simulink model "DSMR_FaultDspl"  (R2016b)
settings: Solver=FixedStepDiscrete  StartTime=0.0  StopTime=10.0  FixedStep=0.02  RelTol=1e-3  EnableMultiTasking=on
undefined symbols (not defined in the file): bin2dec
libraries: simulink x312
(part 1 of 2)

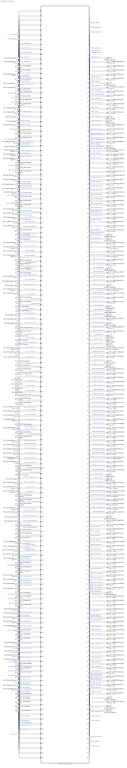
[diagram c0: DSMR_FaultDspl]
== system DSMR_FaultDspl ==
  DFC_CurrRngErr : Inport
  DFC_BattVoltRngErr : Inport  Port=2
  DFC_BattHVMsgTmt : Inport  Port=3
  DFC_BusHVMsgTmt : Inport  Port=4
  DFC_638LinCommErr : Inport  Port=5
  DFC_CellTempTmt : Inport  Port=6
  DFC_CellVoltTmt : Inport  Port=7
  DFC_InCanBusOff : Inport  Port=8
  DFC_VeCanBusOff : Inport  Port=9
  DFC_Msg2A3Tmt : Inport  Port=10
  DFC_RcMsg2A3Mis : Inport  Port=11
  DFC_ChkSumMsg2A3Err : Inport  Port=12
  DFC_RcMsg2A5Mis : Inport  Port=13
  DFC_RcMsg2A7Mis : Inport  Port=14
  DFC_CrashNpl : Inport  Port=15
  DFC_FuseNpl : Inport  Port=16
  DFC_Kl30cVoltLoErr : Inport  Port=17
  DFC_PosStuckMax : Inport  Port=18
  DFC_MPosStuckMin : Inport  Port=19
  DFC_MNegStuckMax : Inport  Port=20
  DFC_MNegStuckMin : Inport  Port=21
  DFC_PrStuckMin : Inport  Port=22
  DFC_DChrgPosStuckMax : Inport  Port=23
  DFC_DChrgPosStuckMin : Inport  Port=24
  DFC_DChrgNegStuckMax : Inport  Port=25
  DFC_DChrgNegStuckMin : Inport  Port=26
  DFC_HvPwrUpFail : Inport  Port=27
  DFC_DChrgPwrUpFail : Inport  Port=28
  DFC_BattTAlrmMax : Inport  Port=29
  DFC_BattTFaultMax : Inport  Port=30
  DFC_BattTAlrmMin : Inport  Port=31
  DFC_BattTFaultMin : Inport  Port=32
  DFC_BattTempVldMin : Inport  Port=33
  DFC_BattTCnstMax : Inport  Port=34
  DFC_BattTGradtMax : Inport  Port=35
  DFC_CellVoltAlrmMax : Inport  Port=36
  DFC_CellVoltFaultMax : Inport  Port=37
  DFC_CellVoltFusfMax : Inport  Port=38
  DFC_CellVoltAlrmMin : Inport  Port=39
  DFC_CellVoltFusfMin : Inport  Port=40
  DFC_CellVoltFaultMin : Inport  Port=41
  DFC_CellVoltVldMin : Inport  Port=42
  DFC_CellVoltNpl : Inport  Port=43
  DFC_Msg2E6Tmt : Inport  Port=44
  DFC_RcMsg2E6Mis : Inport  Port=45
  DFC_ChkSumMsg2E6Err : Inport  Port=46
  DFC_RcMsg2E1Mis : Inport  Port=47
  DFC_ChkSumMsg2E1Err : Inport  Port=48
  DFC_DcCanBusOff : Inport  Port=49
  DFC_DChrgTCnntMax : Inport  Port=50
  DFC_ChrgOCNpl : Inport  Port=51
  DFC_DisChOCNpl : Inport  Port=52
  DFC_BattVoltHiMax : Inport  Port=53
  DFC_BattVoltLoMin : Inport  Port=54
  DFC_ThmRnwy : Inport  Port=55
  DFC_AChrgPortOvrTemp : Inport  Port=56
  DFC_CurrOffsPlaus : Inport  Port=57
  DFC_CurrStukPlaus : Inport  Port=58
  DFC_CurrChrgPlaus : Inport  Port=59
  DFC_BattUNpl : Inport  Port=60
  DFC_BattVoltVld : Inport  Port=61
  DFC_PackUNpl : Inport  Port=62
  DFC_PackVoltVld : Inport  Port=63
  DFC_DChrgUNpl : Inport  Port=64
  DFC_DChrgVoltVld : Inport  Port=65
  DFC_BoardTempTmt : Inport  Port=66
  DFC_HvilMax : Inport  Port=67
  DFC_HvilMin : Inport  Port=68
  DFC_HvilSig : Inport  Port=69
  DFC_ChkSumMsg050Err : Inport  Port=70
  DFC_RcMsg050Mis : Inport  Port=71
  DFC_CrashHwNpl : Inport  Port=72
  DFC_IsoChkLv1 : Inport  Port=73
  DFC_IsoChkLv2 : Inport  Port=74
  DFC_InsResValdFault : Inport  Port=75
  DFC_Kl30OutRngErr : Inport  Port=76
  DFC_Kl30VoltLoErr : Inport  Port=77
  DFC_Kl30VoltHiErr : Inport  Port=78
  DFC_EepReadErr : Inport  Port=79
  DFC_BalStuckMax : Inport  Port=80
  DFC_BalStuckMin : Inport  Port=81
  DFC_CSCPwrSpyHiErr : Inport  Port=82
  DFC_CSCPwrSpyLoErr : Inport  Port=83
  DFC_CmcBordOTMax : Inport  Port=84
  DFC_BattTWarnMax : Inport  Port=85
  DFC_BattTWarnMin : Inport  Port=86
  DFC_BattTempVldMax : Inport  Port=87
  DFC_BattTHopMax : Inport  Port=88
  DFC_CellVoltRngHiErr : Inport  Port=89
  DFC_CellVoltRngLoErr : Inport  Port=90
  DFC_CellVoltWarnMax : Inport  Port=91
  DFC_CellVoltWarnMin : Inport  Port=92
  DFC_CellVoltVldMax : Inport  Port=93
  DFC_AChrgCurrMish : Inport  Port=94
  DFC_DChrgCurrMish : Inport  Port=95
  DFC_DChrgLowTempCurrMish : Inport  Port=96
  DFC_AChrgVoltMish : Inport  Port=97
  DFC_DChrgVoltMish : Inport  Port=98
  DFC_DChrgBattTMin : Inport  Port=99
  DFC_CC2Chk : Inport  Port=100
  DFC_APlusChk : Inport  Port=101
  DFC_DChrgMsgTmt : Inport  Port=102
  DFC_DChrgTNegElecMax : Inport  Port=103
  DFC_DChrgTNegElecMin : Inport  Port=104
  DFC_DChrgTNegElecSig : Inport  Port=105
  DFC_DChrgTPosElecMax : Inport  Port=106
  DFC_DChrgTPosElecMin : Inport  Port=107
  DFC_DChrgTPosElecSig : Inport  Port=108
  DFC_CcuSelfChkErr : Inport  Port=109
  DFC_ChrgOCMin : Inport  Port=110
  DFC_ChrgOCMax : Inport  Port=111
  DFC_DisChOCMin : Inport  Port=112
  DFC_DisChOCMax : Inport  Port=113
  DFC_SocRngLoMax : Inport  Port=114
  DFC_SocRngLoMin : Inport  Port=115
  DFC_SocRngHiMax : Inport  Port=116
  DFC_SocRngHiMin : Inport  Port=117
  DFC_InClntOverTmp : Inport  Port=118
  DFC_OutClntOverTmp : Inport  Port=119
  DFC_ClntDsTElecMax : Inport  Port=120
  DFC_ClntDsTElecMin : Inport  Port=121
  DFC_ClntDsTElecSig : Inport  Port=122
  DFC_ClntUsTElecMax : Inport  Port=123
  DFC_ClntUsTElecMin : Inport  Port=124
  DFC_ClntUsTElecSig : Inport  Port=125
  DFC_CoolPerfPlaus : Inport  Port=126
  DFC_HtgPerfPlaus : Inport  Port=127
  DFC_DChrgFobd : Inport  Port=128
  DFC_DChrgHvOnFail : Inport  Port=129
  DFC_AChgHVOnTmt : Inport  Port=130
  DFC_AChgHVOffTmt : Inport  Port=131
  DFC_AChgS2ClsdTmt : Inport  Port=132
  DFC_DChrgStakeErr : Inport  Port=133
  DFC_DChrgStkVoltErr : Inport  Port=134
  DFC_DChrgStkCurrErr : Inport  Port=135
  DFC_AChgPileRdyTmt : Inport  Port=136
  DFC_DChrgCHMTmt : Inport  Port=137
  DFC_DChrgCRMTmt : Inport  Port=138
  DFC_DChrgCMLTmt : Inport  Port=139
  DFC_DChrgCROTmt : Inport  Port=140
  DFC_DChrgCCSTmt : Inport  Port=141
  DFC_DChrgCSTTmt : Inport  Port=142
  DFC_DChrgCSDTmt : Inport  Port=143
  DFC_DChrgParaChk : Inport  Port=144
  DFC_DChrgCableChk : Inport  Port=145
  DFC_DChrgSLACTOut : Inport  Port=146
  DFC_DChrgCnntErr : Inport  Port=147
  DFC_DChrgLckErr : Inport  Port=148
  DFC_AChrgCnntErr : Inport  Port=149
  DFC_AChgLckTmt : Inport  Port=150
  DFC_AChgRdyPndiTmt : Inport  Port=151
  DFC_AChgRdyTmt : Inport  Port=152
  DFC_AChgingErr : Inport  Port=153
  DFC_AChgUnlckTmt : Inport  Port=154
  DFC_AChgFobd : Inport  Port=155
  DFC_SocValJmp : Inport  Port=156
  BMS_DSMR_FaultDspl : Subsystem
  DSMR_CurrRngErr : Outport
  DSMR_BattVoltRngErr : Outport  Port=2
  DSMR_BattHVMsgTmt : Outport  Port=3
  DSMR_BusHVMsgTmt : Outport  Port=4
  DSMR_638LinCommErr : Outport  Port=5
  DSMR_CellTempTmt : Outport  Port=6
  DSMR_CellVoltTmt : Outport  Port=7
  DSMR_InCanBusOff : Outport  Port=8
  DSMR_VeCanBusOff : Outport  Port=9
  DSMR_Msg2A3Tmt : Outport  Port=10
  DSMR_RcMsg2A3Mis : Outport  Port=11
  DSMR_ChkSumMsg2A3Err : Outport  Port=12
  DSMR_RcMsg2A5Mis : Outport  Port=13
  DSMR_RcMsg2A7Mis : Outport  Port=14
  DSMR_CrashNpl : Outport  Port=15
  DSMR_FuseNpl : Outport  Port=16
  DSMR_Kl30cVoltLoErr : Outport  Port=17
  DSMR_PosStuckMax : Outport  Port=18
  DSMR_MPosStuckMin : Outport  Port=19
  DSMR_MNegStuckMax : Outport  Port=20
  DSMR_MNegStuckMin : Outport  Port=21
  DSMR_PrStuckMin : Outport  Port=22
  DSMR_DChrgPosStuckMax : Outport  Port=23
  DSMR_DChrgPosStuckMin : Outport  Port=24
  DSMR_DChrgNegStuckMax : Outport  Port=25
  DSMR_DChrgNegStuckMin : Outport  Port=26
  DSMR_HvPwrUpFail : Outport  Port=27
  DSMR_DChrgPwrUpFail : Outport  Port=28
  DSMR_BattTAlrmMax : Outport  Port=29
  DSMR_BattTFaultMax : Outport  Port=30
  DSMR_BattTAlrmMin : Outport  Port=31
  DSMR_BattTFaultMin : Outport  Port=32
  DSMR_BattTempVldMin : Outport  Port=33
  DSMR_BattTCnstMax : Outport  Port=34
  DSMR_BattTGradtMax : Outport  Port=35
  DSMR_CellVoltAlrmMax : Outport  Port=36
  DSMR_CellVoltFaultMax : Outport  Port=37
  DSMR_CellVoltFusfMax : Outport  Port=38
  DSMR_CellVoltAlrmMin : Outport  Port=39
  DSMR_CellVoltFusfMin : Outport  Port=40
  DSMR_CellVoltFaultMin : Outport  Port=41
  DSMR_CellVoltVldMin : Outport  Port=42
  DSMR_CellVoltNpl : Outport  Port=43
  DSMR_Obc2E6Tmt : Outport  Port=44
  DSMR_RcMsg2E6Mis : Outport  Port=45
  DSMR_ChkSumMsg2E6Err : Outport  Port=46
  DSMR_RcMsg2E1Mis : Outport  Port=47
  DSMR_ChkSumMsg2E1Err : Outport  Port=48
  DSMR_DcCanBusOff : Outport  Port=49
  DSMR_DChrgTCnntMax : Outport  Port=50
  DSMR_ChrgOCNpl : Outport  Port=51
  DSMR_DisChOCNpl : Outport  Port=52
  DSMR_BattVoltHiMax : Outport  Port=53
  DSMR_BattVoltLoMin : Outport  Port=54
  DSMR_ThmRnwy : Outport  Port=55
  DSMR_AChrgPortOvrTemp : Outport  Port=56
  DSMR_CurrOffsPlaus : Outport  Port=57
  DSMR_CurrStukPlaus : Outport  Port=58
  DSMR_CurrChrgPlaus : Outport  Port=59
  DSMR_BattUNpl : Outport  Port=60
  DSMR_BattVoltVld : Outport  Port=61
  DSMR_PackUNpl : Outport  Port=62
  DSMR_PackVoltVld : Outport  Port=63
  DSMR_DChrgUNpl : Outport  Port=64
  DSMR_DChrgVoltVld : Outport  Port=65
  DSMR_BoardTempTmt : Outport  Port=66
  DSMR_HvilMax : Outport  Port=67
  DSMR_HvilMin : Outport  Port=68
  DSMR_HvilSig : Outport  Port=69
  DSMR_ChkSumMsg050Err : Outport  Port=70
  DSMR_RcMsg050Mis : Outport  Port=71
  DSMR_CrashHwNpl : Outport  Port=72
  DSMR_IsoChkLv1 : Outport  Port=73
  DSMR_IsoChkLv2 : Outport  Port=74
  DSMR_InsResValdFault : Outport  Port=75
  DSMR_Kl30OutRngErr : Outport  Port=76
  DSMR_Kl30VoltLoErr : Outport  Port=77
  DSMR_Kl30VoltHiErr : Outport  Port=78
  DSMR_EepReadErr : Outport  Port=79
  DSMR_BalStuckMax : Outport  Port=80
  DSMR_BalStuckMin : Outport  Port=81
  DSMR_CSCPwrSpyHiErr : Outport  Port=82
  DSMR_CSCPwrSpyLoErr : Outport  Port=83
  DSMR_CmcBordOTMax : Outport  Port=84
  DSMR_BattTWarnMax : Outport  Port=85
  DSMR_BattTWarnMin : Outport  Port=86
  DSMR_BattTempVldMax : Outport  Port=87
  DSMR_BattTHopMax : Outport  Port=88
  DSMR_CellVoltRngHiErr : Outport  Port=89
  DSMR_CellVoltRngLoErr : Outport  Port=90
  DSMR_CellVoltWarnMax : Outport  Port=91
  DSMR_CellVoltWarnMin : Outport  Port=92
  DSMR_CellVoltVldMax : Outport  Port=93
  DSMR_AChrgCurrMish : Outport  Port=94
  DSMR_DChrgCurrMish : Outport  Port=95
  DSMR_DChrgLowTempCurrMish : Outport  Port=96
  DSMR_AChrgVoltMish : Outport  Port=97
  DSMR_DChrgVoltMish : Outport  Port=98
  DSMR_DChrgBattTMin : Outport  Port=99
  DSMR_CC2Chk : Outport  Port=100
  DSMR_APlusChk : Outport  Port=101
  DSMR_DChrgMsgTmt : Outport  Port=102
  DSMR_DChrgTNegElecMax : Outport  Port=103
  DSMR_DChrgTNegElecMin : Outport  Port=104
  DSMR_DChrgTNegElecSig : Outport  Port=105
  DSMR_DChrgTPosElecMax : Outport  Port=106
  DSMR_DChrgTPosElecMin : Outport  Port=107
  DSMR_DChrgTPosElecSig : Outport  Port=108
  DSMR_CcuSelfChkErr : Outport  Port=109
  DSMR_ChrgOCMin : Outport  Port=110
  DSMR_ChrgOCMax : Outport  Port=111
  DSMR_DisChOCMin : Outport  Port=112
  DSMR_DisChOCMax : Outport  Port=113
  DSMR_SocRngLoMax : Outport  Port=114
  DSMR_SocRngLoMin : Outport  Port=115
  DSMR_SocRngHiMax : Outport  Port=116
  DSMR_SocRngHiMin : Outport  Port=117
  DSMR_InClntOverTmp : Outport  Port=118
  DSMR_OutClntOverTmp : Outport  Port=119
  DSMR_ClntDsTElecMax : Outport  Port=120
  DSMR_ClntDsTElecMin : Outport  Port=121
  DSMR_ClntDsTElecSig : Outport  Port=122
  DSMR_ClntUsTElecMax : Outport  Port=123
  DSMR_ClntUsTElecMin : Outport  Port=124
  DSMR_ClntUsTElecSig : Outport  Port=125
  DSMR_CoolPerfPlaus : Outport  Port=126
  DSMR_HtgPerfPlaus : Outport  Port=127
  DSMR_DChrgFobd : Outport  Port=128
  DSMR_DChrgHvOnFail : Outport  Port=129
  DSMR_AChgHVOnTmt : Outport  Port=130
  DSMR_AChgHVOffTmt : Outport  Port=131
  DSMR_AChgS2ClsdTmt : Outport  Port=132
  DSMR_DChrgStakeErr : Outport  Port=133
  DSMR_DChrgStkVoltErr : Outport  Port=134
  DSMR_DChrgStkCurrErr : Outport  Port=135
  DSMR_AChgPileRdyTmt : Outport  Port=136
  DSMR_DChrgCHMTmt : Outport  Port=137
  DSMR_DChrgCRMTmt : Outport  Port=138
  DSMR_DChrgCMLTmt : Outport  Port=139
  DSMR_DChrgCROTmt : Outport  Port=140
  DSMR_DChrgCCSTmt : Outport  Port=141
  DSMR_DChrgCSTTmt : Outport  Port=142
  DSMR_DChrgCSDTmt : Outport  Port=143
  DSMR_DChrgParaChk : Outport  Port=144
  DSMR_DChrgCableChk : Outport  Port=145
  DSMR_DChrgSLACTOut : Outport  Port=146
  DSMR_DChrgCnntErr : Outport  Port=147
  DSMR_DChrgLckErr : Outport  Port=148
  DSMR_AChrgCnntErr : Outport  Port=149
  DSMR_AChgLckTmt : Outport  Port=150
  DSMR_AChgRdyPndiTmt : Outport  Port=151
  DSMR_AChgRdyTmt : Outport  Port=152
  DSMR_AChgingErr : Outport  Port=153
  DSMR_AChgUnlckTmt : Outport  Port=154
  DSMR_AChgFobd : Outport  Port=155
  DSMR_SocValJmp : Outport  Port=156
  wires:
  DFC_CurrRngErr/1 -> BMS_DSMR_FaultDspl/1(DFC_CurrRngErr)  "DFC_CurrRngErr"
  DFC_BattVoltRngErr/1 -> BMS_DSMR_FaultDspl/2(DFC_BattVoltRngErr)  "DFC_BattVoltRngErr"
  DFC_BattHVMsgTmt/1 -> BMS_DSMR_FaultDspl/3(DFC_BattHVMsgTmt)  "DFC_BattHVMsgTmt"
  DFC_BusHVMsgTmt/1 -> BMS_DSMR_FaultDspl/4(DFC_BusHVMsgTmt)  "DFC_BusHVMsgTmt"
  DFC_638LinCommErr/1 -> BMS_DSMR_FaultDspl/5(DFC_638LinCommErr)  "DFC_638LinCommErr"
  DFC_CellTempTmt/1 -> BMS_DSMR_FaultDspl/6(DFC_CellTempTmt)  "DFC_CellTempTmt"
  DFC_CellVoltTmt/1 -> BMS_DSMR_FaultDspl/7(DFC_CellVoltTmt)  "DFC_CellVoltTmt"
  DFC_InCanBusOff/1 -> BMS_DSMR_FaultDspl/8(DFC_InCanBusOff)  "DFC_InCanBusOff"
  DFC_VeCanBusOff/1 -> BMS_DSMR_FaultDspl/9(DFC_VeCanBusOff)  "DFC_VeCanBusOff"
  DFC_Msg2A3Tmt/1 -> BMS_DSMR_FaultDspl/10(DFC_Msg2A3Tmt)  "DFC_Msg2A3Tmt"
  DFC_RcMsg2A3Mis/1 -> BMS_DSMR_FaultDspl/11(DFC_RcMsg2A3Mis)  "DFC_RcMsg2A3Mis"
  DFC_ChkSumMsg2A3Err/1 -> BMS_DSMR_FaultDspl/12(DFC_ChkSumMsg2A3Err)  "DFC_ChkSumMsg2A3Err"
  DFC_RcMsg2A5Mis/1 -> BMS_DSMR_FaultDspl/13(DFC_RcMsg2A5Mis)  "DFC_RcMsg2A5Mis"
  DFC_RcMsg2A7Mis/1 -> BMS_DSMR_FaultDspl/14(DFC_RcMsg2A7Mis)  "DFC_RcMsg2A7Mis"
  DFC_CrashNpl/1 -> BMS_DSMR_FaultDspl/15(DFC_CrashNpl)  "DFC_CrashNpl"
  DFC_FuseNpl/1 -> BMS_DSMR_FaultDspl/16(DFC_FuseNpl)  "DFC_FuseNpl"
  DFC_Kl30cVoltLoErr/1 -> BMS_DSMR_FaultDspl/17(DFC_Kl30cVoltLoErr)  "DFC_Kl30cVoltLoErr"
  DFC_PosStuckMax/1 -> BMS_DSMR_FaultDspl/18(DFC_PosStuckMax)  "DFC_PosStuckMax"
  DFC_MPosStuckMin/1 -> BMS_DSMR_FaultDspl/19(DFC_MPosStuckMin)  "DFC_MPosStuckMin"
  DFC_MNegStuckMax/1 -> BMS_DSMR_FaultDspl/20(DFC_MNegStuckMax)  "DFC_MNegStuckMax"
  DFC_MNegStuckMin/1 -> BMS_DSMR_FaultDspl/21(DFC_MNegStuckMin)  "DFC_MNegStuckMin"
  DFC_PrStuckMin/1 -> BMS_DSMR_FaultDspl/22(DFC_PrStuckMin)  "DFC_PrStuckMin"
  DFC_DChrgPosStuckMax/1 -> BMS_DSMR_FaultDspl/23(DFC_DChrgPosStuckMax)  "DFC_DChrgPosStuckMax"
  DFC_DChrgPosStuckMin/1 -> BMS_DSMR_FaultDspl/24(DFC_DChrgPosStuckMin)  "DFC_DChrgPosStuckMin"
  DFC_DChrgNegStuckMax/1 -> BMS_DSMR_FaultDspl/25(DFC_DChrgNegStuckMax)  "DFC_DChrgNegStuckMax"
  DFC_DChrgNegStuckMin/1 -> BMS_DSMR_FaultDspl/26(DFC_DChrgNegStuckMin)  "DFC_DChrgNegStuckMin"
  DFC_HvPwrUpFail/1 -> BMS_DSMR_FaultDspl/27(DFC_HvPwrUpFail)  "DFC_HvPwrUpFail"
  DFC_DChrgPwrUpFail/1 -> BMS_DSMR_FaultDspl/28(DFC_DChrgPwrUpFail)  "DFC_DChrgPwrUpFail"
  DFC_BattTAlrmMax/1 -> BMS_DSMR_FaultDspl/29(DFC_BattTAlrmMax)  "DFC_BattTAlrmMax"
  DFC_BattTFaultMax/1 -> BMS_DSMR_FaultDspl/30(DFC_BattTFaultMax)  "DFC_BattTFaultMax"
  DFC_BattTAlrmMin/1 -> BMS_DSMR_FaultDspl/31(DFC_BattTAlrmMin)  "DFC_BattTAlrmMin"
  DFC_BattTFaultMin/1 -> BMS_DSMR_FaultDspl/32(DFC_BattTFaultMin)  "DFC_BattTFaultMin"
  DFC_BattTempVldMin/1 -> BMS_DSMR_FaultDspl/33(DFC_BattTempVldMin)  "DFC_BattTempVldMin"
  DFC_BattTCnstMax/1 -> BMS_DSMR_FaultDspl/34(DFC_BattTCnstMax)  "DFC_BattTCnstMax"
  DFC_BattTGradtMax/1 -> BMS_DSMR_FaultDspl/35(DFC_BattTGradtMax)  "DFC_BattTGradtMax"
  DFC_CellVoltAlrmMax/1 -> BMS_DSMR_FaultDspl/36(DFC_CellVoltAlrmMax)  "DFC_CellVoltAlrmMax"
  DFC_CellVoltFaultMax/1 -> BMS_DSMR_FaultDspl/37(DFC_CellVoltFaultMax)  "DFC_CellVoltFaultMax"
  DFC_CellVoltFusfMax/1 -> BMS_DSMR_FaultDspl/38(DFC_CellVoltFusfMax)  "DFC_CellVoltFusfMax"
  DFC_CellVoltAlrmMin/1 -> BMS_DSMR_FaultDspl/39(DFC_CellVoltAlrmMin)  "DFC_CellVoltAlrmMin"
  DFC_CellVoltFusfMin/1 -> BMS_DSMR_FaultDspl/40(DFC_CellVoltFusfMin)  "DFC_CellVoltFusfMin"
  DFC_CellVoltFaultMin/1 -> BMS_DSMR_FaultDspl/41(DFC_CellVoltFaultMin)  "DFC_CellVoltFaultMin"
  DFC_CellVoltVldMin/1 -> BMS_DSMR_FaultDspl/42(DFC_CellVoltVldMin)  "DFC_CellVoltVldMin"
  DFC_CellVoltNpl/1 -> BMS_DSMR_FaultDspl/43(DFC_CellVoltNpl)  "DFC_CellVoltNpl"
  DFC_Msg2E6Tmt/1 -> BMS_DSMR_FaultDspl/44(DFC_Msg2E6Tmt)  "DFC_Msg2E6Tmt"
  DFC_RcMsg2E6Mis/1 -> BMS_DSMR_FaultDspl/45(DFC_RcMsg2E6Mis)  "DFC_RcMsg2E0Mis"
  DFC_ChkSumMsg2E6Err/1 -> BMS_DSMR_FaultDspl/46(DFC_ChkSumMsg2E6Err)  "DFC_ChkSumMsg2E0Err"
  DFC_RcMsg2E1Mis/1 -> BMS_DSMR_FaultDspl/47(DFC_RcMsg2E1Mis)  "DFC_RcMsg2E1Mis"
  DFC_ChkSumMsg2E1Err/1 -> BMS_DSMR_FaultDspl/48(DFC_ChkSumMsg2E1Err)  "DFC_ChkSumMsg2E1Err"
  DFC_DcCanBusOff/1 -> BMS_DSMR_FaultDspl/49(DFC_DcCanBusOff)  "DFC_DcCanBusOff"
  DFC_DChrgTCnntMax/1 -> BMS_DSMR_FaultDspl/50(DFC_DChrgTCnntMax)  "DFC_DChrgTCnntMax"
  DFC_ChrgOCNpl/1 -> BMS_DSMR_FaultDspl/51(DFC_ChrgOCNpl)  "DFC_ChrgOCNpl"
  DFC_DisChOCNpl/1 -> BMS_DSMR_FaultDspl/52(DFC_DisChOCNpl)  "DFC_DisChOCNpl"
  DFC_BattVoltHiMax/1 -> BMS_DSMR_FaultDspl/53(DFC_BattVoltHiMax)  "DFC_BattVoltHiMax"
  DFC_BattVoltLoMin/1 -> BMS_DSMR_FaultDspl/54(DFC_BattVoltLoMin)  "DFC_BattVoltLoMin"
  DFC_ThmRnwy/1 -> BMS_DSMR_FaultDspl/55(DFC_ThmRnwy)  "DFC_ThmRnwy"
  DFC_AChrgPortOvrTemp/1 -> BMS_DSMR_FaultDspl/56(DFC_AChrgPortOvrTemp)  "DFC_AChrgPortOvrTemp"
  DFC_CurrOffsPlaus/1 -> BMS_DSMR_FaultDspl/57(DFC_CurrOffsPlaus)  "DFC_CurrOffsPlaus"
  DFC_CurrStukPlaus/1 -> BMS_DSMR_FaultDspl/58(DFC_CurrStukPlaus)  "DFC_CurrStukPlaus"
  DFC_CurrChrgPlaus/1 -> BMS_DSMR_FaultDspl/59(DFC_CurrChrgPlaus)  "DFC_CurrChrgPlaus"
  DFC_BattUNpl/1 -> BMS_DSMR_FaultDspl/60(DFC_BattUNpl)  "DFC_BattUNpl"
  DFC_BattVoltVld/1 -> BMS_DSMR_FaultDspl/61(DFC_BattVoltVld)  "DFC_BattVoltVld"
  DFC_PackUNpl/1 -> BMS_DSMR_FaultDspl/62(DFC_PackUNpl)  "DFC_PackUNpl"
  DFC_PackVoltVld/1 -> BMS_DSMR_FaultDspl/63(DFC_PackVoltVld)  "DFC_PackVoltVld"
  DFC_DChrgUNpl/1 -> BMS_DSMR_FaultDspl/64(DFC_DChrgUNpl)  "DFC_DChrgUNpl"
  DFC_DChrgVoltVld/1 -> BMS_DSMR_FaultDspl/65(DFC_DChrgVoltVld)  "DFC_DChrgVoltVld"
  DFC_BoardTempTmt/1 -> BMS_DSMR_FaultDspl/66(DFC_BoardTempTmt)  "DFC_BoardTempTmt"
  DFC_HvilMax/1 -> BMS_DSMR_FaultDspl/67(DFC_HvilMax)  "DFC_HvilMax"
  DFC_HvilMin/1 -> BMS_DSMR_FaultDspl/68(DFC_HvilMin)  "DFC_HvilMin"
  DFC_HvilSig/1 -> BMS_DSMR_FaultDspl/69(DFC_HvilSig)  "DFC_HvilSig"
  DFC_ChkSumMsg050Err/1 -> BMS_DSMR_FaultDspl/70(DFC_ChkSumMsg050Err)  "DFC_ChkSumMsg050Err"
  DFC_RcMsg050Mis/1 -> BMS_DSMR_FaultDspl/71(DFC_RcMsg050Mis)  "DFC_RcMsg050Mis"
  DFC_CrashHwNpl/1 -> BMS_DSMR_FaultDspl/72(DFC_CrashHwNpl)  "DFC_CrashHwNpl"
  DFC_IsoChkLv1/1 -> BMS_DSMR_FaultDspl/73(DFC_IsoChkLv1)  "DFC_IsoChkLv1"
  DFC_IsoChkLv2/1 -> BMS_DSMR_FaultDspl/74(DFC_IsoChkLv2)  "DFC_IsoChkLv2"
  DFC_InsResValdFault/1 -> BMS_DSMR_FaultDspl/75(DFC_InsResValdFault)  "DFC_InsResValdFault"
  DFC_Kl30OutRngErr/1 -> BMS_DSMR_FaultDspl/76(DFC_Kl30OutRngErr)  "DFC_Kl30OutRngErr"
  DFC_Kl30VoltLoErr/1 -> BMS_DSMR_FaultDspl/77(DFC_Kl30VoltLoErr)  "DFC_Kl30VoltLoErr"
  DFC_Kl30VoltHiErr/1 -> BMS_DSMR_FaultDspl/78(DFC_Kl30VoltHiErr)  "DFC_Kl30VoltHiErr"
  DFC_EepReadErr/1 -> BMS_DSMR_FaultDspl/79(DFC_EepReadErr)  "DFC_EepReadErr"
  DFC_BalStuckMax/1 -> BMS_DSMR_FaultDspl/80(DFC_BalStuckMax)  "DFC_BalStuckMax"
  DFC_BalStuckMin/1 -> BMS_DSMR_FaultDspl/81(DFC_BalStuckMin)  "DFC_BalStuckMin"
  DFC_CSCPwrSpyHiErr/1 -> BMS_DSMR_FaultDspl/82(DFC_CSCPwrSpyHiErr)  "DFC_CSCPwrSpyHiErr"
  DFC_CSCPwrSpyLoErr/1 -> BMS_DSMR_FaultDspl/83(DFC_CSCPwrSpyLoErr)  "DFC_CSCPwrSpyLoErr"
  DFC_CmcBordOTMax/1 -> BMS_DSMR_FaultDspl/84(DFC_CmcBordOTMax)  "DFC_CmcBordOTMax"
  DFC_BattTWarnMax/1 -> BMS_DSMR_FaultDspl/85(DFC_BattTWarnMax)  "DFC_BattTWarnMax"
  DFC_BattTWarnMin/1 -> BMS_DSMR_FaultDspl/86(DFC_BattTWarnMin)  "DFC_BattTWarnMin"
  DFC_BattTempVldMax/1 -> BMS_DSMR_FaultDspl/87(DFC_BattTempVldMax)  "DFC_BattTempVldMax"
  DFC_BattTHopMax/1 -> BMS_DSMR_FaultDspl/88(DFC_BattTHopMax)  "DFC_BattTHopMax"
  DFC_CellVoltRngHiErr/1 -> BMS_DSMR_FaultDspl/89(DFC_CellVoltRngHiErr)  "DFC_CellVoltRngHiErr"
  DFC_CellVoltRngLoErr/1 -> BMS_DSMR_FaultDspl/90(DFC_CellVoltRngLoErr)  "DFC_CellVoltRngLoErr"
  DFC_CellVoltWarnMax/1 -> BMS_DSMR_FaultDspl/91(DFC_CellVoltWarnMax)  "DFC_CellVoltWarnMax"
  DFC_CellVoltWarnMin/1 -> BMS_DSMR_FaultDspl/92(DFC_CellVoltWarnMin)  "DFC_CellVoltWarnMin"
  DFC_CellVoltVldMax/1 -> BMS_DSMR_FaultDspl/93(DFC_CellVoltVldMax)  "DFC_CellVoltVldMax"
  DFC_AChrgCurrMish/1 -> BMS_DSMR_FaultDspl/94(DFC_AChrgCurrMish)  "DFC_AChrgCurrMish"
  DFC_DChrgCurrMish/1 -> BMS_DSMR_FaultDspl/95(DFC_DChrgCurrMish)  "DFC_DChrgCurrMish"
  DFC_DChrgLowTempCurrMish/1 -> BMS_DSMR_FaultDspl/96(DFC_DChrgLowTempCurrMish)  "DFC_DChrgLowTempCurrMish"
  DFC_AChrgVoltMish/1 -> BMS_DSMR_FaultDspl/97(DFC_AChrgVoltMish)  "DFC_AChrgVoltMish"
  DFC_DChrgVoltMish/1 -> BMS_DSMR_FaultDspl/98(DFC_DChrgVoltMish)  "DFC_DChrgVoltMish"
  DFC_DChrgBattTMin/1 -> BMS_DSMR_FaultDspl/99(DFC_DChrgBattTMin)  "DFC_DChrgBattTMin"
  DFC_CC2Chk/1 -> BMS_DSMR_FaultDspl/100(DFC_CC2Chk)  "DFC_CC2Chk"
  DFC_APlusChk/1 -> BMS_DSMR_FaultDspl/101(DFC_APlusChk)  "DFC_APlusChk"
  DFC_DChrgMsgTmt/1 -> BMS_DSMR_FaultDspl/102(DFC_DChrgMsgTmt)  "DFC_DChrgMsgTmt"
  DFC_DChrgTNegElecMax/1 -> BMS_DSMR_FaultDspl/103(DFC_DChrgTNegElecMax)  "DFC_DChrgTNegElecMax"
  DFC_DChrgTNegElecMin/1 -> BMS_DSMR_FaultDspl/104(DFC_DChrgTNegElecMin)  "DFC_DChrgTNegElecMin"
  DFC_DChrgTNegElecSig/1 -> BMS_DSMR_FaultDspl/105(DFC_DChrgTNegElecSig)  "DFC_DChrgTNegElecSig"
  DFC_DChrgTPosElecMax/1 -> BMS_DSMR_FaultDspl/106(DFC_DChrgTPosElecMax)  "DFC_DChrgTPosElecMax"
  DFC_DChrgTPosElecMin/1 -> BMS_DSMR_FaultDspl/107(DFC_DChrgTPosElecMin)  "DFC_DChrgTPosElecMin"
  DFC_DChrgTPosElecSig/1 -> BMS_DSMR_FaultDspl/108(DFC_DChrgTPosElecSig)  "DFC_DChrgTPosElecSig"
  DFC_CcuSelfChkErr/1 -> BMS_DSMR_FaultDspl/109(DFC_CcuSelfChkErr)  "DFC_CcuSelfChkErr"
  DFC_ChrgOCMin/1 -> BMS_DSMR_FaultDspl/110(DFC_ChrgOCMin)  "DFC_ChrgOCMin"
  DFC_ChrgOCMax/1 -> BMS_DSMR_FaultDspl/111(DFC_ChrgOCMax)  "DFC_ChrgOCMax"
  DFC_DisChOCMin/1 -> BMS_DSMR_FaultDspl/112(DFC_DisChOCMin)  "DFC_DisChOCMin"
  DFC_DisChOCMax/1 -> BMS_DSMR_FaultDspl/113(DFC_DisChOCMax)  "DFC_DisChOCMax"
  DFC_SocRngLoMax/1 -> BMS_DSMR_FaultDspl/114(DFC_SocRngLoMax)  "DFC_SocRngLoMax"
  DFC_SocRngLoMin/1 -> BMS_DSMR_FaultDspl/115(DFC_SocRngLoMin)  "DFC_SocRngLoMin"
  DFC_SocRngHiMax/1 -> BMS_DSMR_FaultDspl/116(DFC_SocRngHiMax)  "DFC_SocRngHiMax"
  DFC_SocRngHiMin/1 -> BMS_DSMR_FaultDspl/117(DFC_SocRngHiMin)  "DFC_SocRngHiMin"
  DFC_InClntOverTmp/1 -> BMS_DSMR_FaultDspl/118(DFC_InClntOverTmp)  "DFC_InClntOverTmp"
  DFC_OutClntOverTmp/1 -> BMS_DSMR_FaultDspl/119(DFC_OutClntOverTmp)  "DFC_OutClntOverTmp"
  DFC_ClntDsTElecMax/1 -> BMS_DSMR_FaultDspl/120(DFC_ClntDsTElecMax)  "DFC_ClntDsTElecMax"
  DFC_ClntDsTElecMin/1 -> BMS_DSMR_FaultDspl/121(DFC_ClntDsTElecMin)  "DFC_ClntDsTElecMin"
  DFC_ClntDsTElecSig/1 -> BMS_DSMR_FaultDspl/122(DFC_ClntDsTElecSig)  "DFC_ClntDsTElecSig"
  DFC_ClntUsTElecMax/1 -> BMS_DSMR_FaultDspl/123(DFC_ClntUsTElecMax)  "DFC_ClntUsTElecMax"
  DFC_ClntUsTElecMin/1 -> BMS_DSMR_FaultDspl/124(DFC_ClntUsTElecMin)  "DFC_ClntUsTElecMin"
  DFC_ClntUsTElecSig/1 -> BMS_DSMR_FaultDspl/125(DFC_ClntUsTElecSig)  "DFC_ClntUsTElecSig"
  DFC_CoolPerfPlaus/1 -> BMS_DSMR_FaultDspl/126(DFC_CoolPerfPlaus)  "DFC_CoolPerfPlaus"
  DFC_HtgPerfPlaus/1 -> BMS_DSMR_FaultDspl/127(DFC_HtgPerfPlaus)  "DFC_HtgPerfPlaus"
  DFC_DChrgFobd/1 -> BMS_DSMR_FaultDspl/128(DFC_DChrgFobd)  "DFC_DChrgFobd"
  DFC_DChrgHvOnFail/1 -> BMS_DSMR_FaultDspl/129(DFC_DChrgHvOnFail)  "DFC_DChrgHvOnFail"
  DFC_AChgHVOnTmt/1 -> BMS_DSMR_FaultDspl/130(DFC_AChgHVOnTmt)  "DFC_AChgHVOnTmt"
  DFC_AChgHVOffTmt/1 -> BMS_DSMR_FaultDspl/131(DFC_AChgHVOffTmt)  "DFC_AChgHVOffTmt"
  DFC_AChgS2ClsdTmt/1 -> BMS_DSMR_FaultDspl/132(DFC_AChgS2ClsdTmt)  "DFC_AChgS2ClsdTmt"
  DFC_DChrgStakeErr/1 -> BMS_DSMR_FaultDspl/133(DFC_DChrgStakeErr)  "DFC_DChrgStakeErr"
  DFC_DChrgStkVoltErr/1 -> BMS_DSMR_FaultDspl/134(DFC_DChrgStkVoltErr)  "DFC_DChrgStkVoltErr"
  DFC_DChrgStkCurrErr/1 -> BMS_DSMR_FaultDspl/135(DFC_DChrgStkCurrErr)  "DFC_DChrgStkCurrErr"
  DFC_AChgPileRdyTmt/1 -> BMS_DSMR_FaultDspl/136(DFC_AChgPileRdyTmt)  "DFC_AChgPileRdyTmt"
  DFC_DChrgCHMTmt/1 -> BMS_DSMR_FaultDspl/137(DFC_DChrgCHMTmt)  "DFC_DChrgCHMTmt"
  DFC_DChrgCRMTmt/1 -> BMS_DSMR_FaultDspl/138(DFC_DChrgCRMTmt)  "DFC_DChrgCRMTmt"
  DFC_DChrgCMLTmt/1 -> BMS_DSMR_FaultDspl/139(DFC_DChrgCMLTmt)  "DFC_DChrgCMLTmt"
  DFC_DChrgCROTmt/1 -> BMS_DSMR_FaultDspl/140(DFC_DChrgCROTmt)  "DFC_DChrgCROTmt"
  DFC_DChrgCCSTmt/1 -> BMS_DSMR_FaultDspl/141(DFC_DChrgCCSTmt)  "DFC_DChrgCCSTmt"
  DFC_DChrgCSTTmt/1 -> BMS_DSMR_FaultDspl/142(DFC_DChrgCSTTmt)  "DFC_DChrgCSTTmt"
  DFC_DChrgCSDTmt/1 -> BMS_DSMR_FaultDspl/143(DFC_DChrgCSDTmt)  "DFC_DChrgCSDTmt"
  DFC_DChrgParaChk/1 -> BMS_DSMR_FaultDspl/144(DFC_DChrgParaChk)  "DFC_DChrgParaChk"
  DFC_DChrgCableChk/1 -> BMS_DSMR_FaultDspl/145(DFC_DChrgCableChk)  "DFC_DChrgCableChk"
  DFC_DChrgSLACTOut/1 -> BMS_DSMR_FaultDspl/146(DFC_DChrgSLACTOut)  "DFC_DChrgSLACTOut"
  DFC_DChrgCnntErr/1 -> BMS_DSMR_FaultDspl/147(DFC_DChrgCnntErr)  "DFC_DChrgCnntErr"
  DFC_DChrgLckErr/1 -> BMS_DSMR_FaultDspl/148(DFC_DChrgLckErr)  "DFC_DChrgLckErr"
  DFC_AChrgCnntErr/1 -> BMS_DSMR_FaultDspl/149(DFC_AChrgCnntErr)  "DFC_AChrgCnntErr"
  DFC_AChgLckTmt/1 -> BMS_DSMR_FaultDspl/150(DFC_AChgLckTmt)  "DFC_AChgLckTmt"
  DFC_AChgRdyPndiTmt/1 -> BMS_DSMR_FaultDspl/151(DFC_AChgRdyPndiTmt)  "DFC_AChgRdyPndiTmt"
  DFC_AChgRdyTmt/1 -> BMS_DSMR_FaultDspl/152(DFC_AChgRdyTmt)  "DFC_AChgRdyTmt"
  DFC_AChgingErr/1 -> BMS_DSMR_FaultDspl/153(DFC_AChgingErr)  "DFC_AChgingErr"
  DFC_AChgUnlckTmt/1 -> BMS_DSMR_FaultDspl/154(DFC_AChgUnlckTmt)  "DFC_AChgUnlckTmt"
  DFC_AChgFobd/1 -> BMS_DSMR_FaultDspl/155(DFC_AChgFobd)  "DFC_AChgFobd"
  DFC_SocValJmp/1 -> BMS_DSMR_FaultDspl/156(DFC_SocValJmp)  "DFC_SocValJmp"
  BMS_DSMR_FaultDspl/1(DSMR_CurrRngErr) -> DSMR_CurrRngErr/1  "DSMR_CurrRngErr"
  BMS_DSMR_FaultDspl/2(DSMR_BattVoltRngErr) -> DSMR_BattVoltRngErr/1  "DSMR_BattVoltRngErr"
  BMS_DSMR_FaultDspl/3(DSMR_BattHVMsgTmt) -> DSMR_BattHVMsgTmt/1  "DSMR_BattHVMsgTmt"
  BMS_DSMR_FaultDspl/4(DSMR_BusHVMsgTmt) -> DSMR_BusHVMsgTmt/1  "DSMR_BusHVMsgTmt"
  BMS_DSMR_FaultDspl/5(DSMR_638LinCommErr) -> DSMR_638LinCommErr/1  "DSMR_638LinCommErr"
  BMS_DSMR_FaultDspl/6(DSMR_CellTempTmt) -> DSMR_CellTempTmt/1  "DSMR_CellTempTmt"
  BMS_DSMR_FaultDspl/7(DSMR_CellVoltTmt) -> DSMR_CellVoltTmt/1  "DSMR_CellVoltTmt"
  BMS_DSMR_FaultDspl/8(DSMR_InCanBusOff) -> DSMR_InCanBusOff/1  "DSMR_InCanBusOff"
  BMS_DSMR_FaultDspl/9(DSMR_VeCanBusOff) -> DSMR_VeCanBusOff/1  "DSMR_VeCanBusOff"
  BMS_DSMR_FaultDspl/10(DSMR_Msg2A3Tmt) -> DSMR_Msg2A3Tmt/1  "DSMR_Msg2A3Tmt"
  BMS_DSMR_FaultDspl/11(DSMR_RcMsg2A3Mis) -> DSMR_RcMsg2A3Mis/1  "DSMR_RcMsg2A3Mis"
  BMS_DSMR_FaultDspl/12(DSMR_ChkSumMsg2A3Err) -> DSMR_ChkSumMsg2A3Err/1  "DSMR_ChkSumMsg2A3Err"
  BMS_DSMR_FaultDspl/13(DSMR_RcMsg2A5Mis) -> DSMR_RcMsg2A5Mis/1  "DSMR_RcMsg2A5Mis"
  BMS_DSMR_FaultDspl/14(DSMR_RcMsg2A7Mis) -> DSMR_RcMsg2A7Mis/1  "DSMR_RcMsg2A7Mis"
  BMS_DSMR_FaultDspl/15(DSMR_CrashNpl) -> DSMR_CrashNpl/1  "DSMR_CrashNpl"
  BMS_DSMR_FaultDspl/16(DSMR_FuseNpl) -> DSMR_FuseNpl/1  "DSMR_FuseNpl"
  BMS_DSMR_FaultDspl/17(DSMR_Kl30cVoltLoErr) -> DSMR_Kl30cVoltLoErr/1  "DSMR_Kl30cVoltLoErr"
  BMS_DSMR_FaultDspl/18(DSMR_PosStuckMax) -> DSMR_PosStuckMax/1  "DSMR_PosStuckMax"
  BMS_DSMR_FaultDspl/19(DSMR_MPosStuckMin) -> DSMR_MPosStuckMin/1  "DSMR_MPosStuckMin"
  BMS_DSMR_FaultDspl/20(DSMR_MNegStuckMax) -> DSMR_MNegStuckMax/1  "DSMR_MNegStuckMax"
  BMS_DSMR_FaultDspl/21(DSMR_MNegStuckMin) -> DSMR_MNegStuckMin/1  "DSMR_MNegStuckMin"
  BMS_DSMR_FaultDspl/22(DSMR_PrStuckMin) -> DSMR_PrStuckMin/1  "DSMR_PrStuckMin"
  BMS_DSMR_FaultDspl/23(DSMR_DChrgPosStuckMax) -> DSMR_DChrgPosStuckMax/1  "DSMR_DChrgPosStuckMax"
  BMS_DSMR_FaultDspl/24(DSMR_DChrgPosStuckMin) -> DSMR_DChrgPosStuckMin/1  "DSMR_DChrgPosStuckMin"
  BMS_DSMR_FaultDspl/25(DSMR_DChrgNegStuckMax) -> DSMR_DChrgNegStuckMax/1  "DSMR_DChrgNegStuckMax"
  BMS_DSMR_FaultDspl/26(DSMR_DChrgNegStuckMin) -> DSMR_DChrgNegStuckMin/1  "DSMR_DChrgNegStuckMin"
  BMS_DSMR_FaultDspl/27(DSMR_HvPwrUpFail) -> DSMR_HvPwrUpFail/1  "DSMR_HvPwrUpFail"
  BMS_DSMR_FaultDspl/28(DSMR_DChrgPwrUpFail) -> DSMR_DChrgPwrUpFail/1  "DSMR_DChrgPwrUpFail"
  BMS_DSMR_FaultDspl/29(DSMR_BattTAlrmMax) -> DSMR_BattTAlrmMax/1  "DSMR_BattTAlrmMax"
  BMS_DSMR_FaultDspl/30(DSMR_BattTFaultMax) -> DSMR_BattTFaultMax/1  "DSMR_BattTFaultMax"
  BMS_DSMR_FaultDspl/31(DSMR_BattTAlrmMin) -> DSMR_BattTAlrmMin/1  "DSMR_BattTAlrmMin"
  BMS_DSMR_FaultDspl/32(DSMR_BattTFaultMin) -> DSMR_BattTFaultMin/1  "DSMR_BattTFaultMin"
  BMS_DSMR_FaultDspl/33(DSMR_BattTempVldMin) -> DSMR_BattTempVldMin/1  "DSMR_BattTempVldMin"
  BMS_DSMR_FaultDspl/34(DSMR_BattTCnstMax) -> DSMR_BattTCnstMax/1  "DSMR_BattTCnstMax"
  BMS_DSMR_FaultDspl/35(DSMR_BattTGradtMax) -> DSMR_BattTGradtMax/1  "DSMR_BattTGradtMax"
  BMS_DSMR_FaultDspl/36(DSMR_CellVoltAlrmMax) -> DSMR_CellVoltAlrmMax/1  "DSMR_CellVoltAlrmMax"
  BMS_DSMR_FaultDspl/37(DSMR_CellVoltFaultMax) -> DSMR_CellVoltFaultMax/1  "DSMR_CellVoltFaultMax"
  BMS_DSMR_FaultDspl/38(DSMR_CellVoltFusfMax) -> DSMR_CellVoltFusfMax/1  "DSMR_CellVoltFusfMax"
  BMS_DSMR_FaultDspl/39(DSMR_CellVoltAlrmMin) -> DSMR_CellVoltAlrmMin/1  "DSMR_CellVoltAlrmMin"
  BMS_DSMR_FaultDspl/40(DSMR_CellVoltFusfMin) -> DSMR_CellVoltFusfMin/1  "DSMR_CellVoltFusfMin"
  BMS_DSMR_FaultDspl/41(DSMR_CellVoltFaultMin) -> DSMR_CellVoltFaultMin/1  "DSMR_CellVoltFaultMin"
  BMS_DSMR_FaultDspl/42(DSMR_CellVoltVldMin) -> DSMR_CellVoltVldMin/1  "DSMR_CellVoltVldMin"
  BMS_DSMR_FaultDspl/43(DSMR_CellVoltNpl) -> DSMR_CellVoltNpl/1  "DSMR_CellVoltNpl"
  BMS_DSMR_FaultDspl/44(DSMR_Msg2E6Tmt) -> DSMR_Obc2E6Tmt/1  "DSMR_Msg2E6Tmt"
  BMS_DSMR_FaultDspl/45(DSMR_RcMsg2E6Mis) -> DSMR_RcMsg2E6Mis/1  "DSMR_RcMsg2E0Mis"
  BMS_DSMR_FaultDspl/46(DSMR_ChkSumMsg2E6Err) -> DSMR_ChkSumMsg2E6Err/1  "DSMR_ChkSumMsg2E0Err"
  BMS_DSMR_FaultDspl/47(DSMR_RcMsg2E1Mis) -> DSMR_RcMsg2E1Mis/1  "DSMR_RcMsg2E1Mis"
  BMS_DSMR_FaultDspl/48(DSMR_ChkSumMsg2E1Err) -> DSMR_ChkSumMsg2E1Err/1  "DSMR_ChkSumMsg2E1Err"
  BMS_DSMR_FaultDspl/49(DSMR_DcCanBusOff) -> DSMR_DcCanBusOff/1  "DSMR_DcCanBusOff"
  BMS_DSMR_FaultDspl/50(DSMR_DChrgTCnntMax) -> DSMR_DChrgTCnntMax/1  "DSMR_DChrgTCnntMax"
  BMS_DSMR_FaultDspl/51(DSMR_ChrgOCNpl) -> DSMR_ChrgOCNpl/1  "DSMR_ChrgOCNpl"
  BMS_DSMR_FaultDspl/52(DSMR_DisChOCNpl) -> DSMR_DisChOCNpl/1  "DSMR_DisChOCNpl"
  BMS_DSMR_FaultDspl/53(DSMR_BattVoltHiMax) -> DSMR_BattVoltHiMax/1  "DSMR_BattVoltHiMax"
  BMS_DSMR_FaultDspl/54(DSMR_BattVoltLoMin) -> DSMR_BattVoltLoMin/1  "DSMR_BattVoltLoMin"
  BMS_DSMR_FaultDspl/55(DSMR_ThmRnwy) -> DSMR_ThmRnwy/1  "DSMR_ThmRnwy"
  BMS_DSMR_FaultDspl/56(DSMR_AChrgPortOvrTemp) -> DSMR_AChrgPortOvrTemp/1  "DSMR_AChrgPortOvrTemp"
  BMS_DSMR_FaultDspl/57(DSMR_CurrOffsPlaus) -> DSMR_CurrOffsPlaus/1  "DSMR_CurrOffsPlaus"
  BMS_DSMR_FaultDspl/58(DSMR_CurrStukPlaus) -> DSMR_CurrStukPlaus/1  "DSMR_CurrStukPlaus"
  BMS_DSMR_FaultDspl/59(DSMR_CurrChrgPlaus) -> DSMR_CurrChrgPlaus/1  "DSMR_CurrChrgPlaus"
  BMS_DSMR_FaultDspl/60(DSMR_BattUNpl) -> DSMR_BattUNpl/1  "DSMR_BattUNpl"
  BMS_DSMR_FaultDspl/61(DSMR_BattVoltVld) -> DSMR_BattVoltVld/1  "DSMR_BattVoltVld"
  BMS_DSMR_FaultDspl/62(DSMR_PackUNpl) -> DSMR_PackUNpl/1  "DSMR_PackUNpl"
  BMS_DSMR_FaultDspl/63(DSMR_PackVoltVld) -> DSMR_PackVoltVld/1  "DSMR_PackVoltVld"
  BMS_DSMR_FaultDspl/64(DSMR_DChrgUNpl) -> DSMR_DChrgUNpl/1  "DSMR_DChrgUNpl"
  BMS_DSMR_FaultDspl/65(DSMR_DChrgVoltVld) -> DSMR_DChrgVoltVld/1  "DSMR_DChrgVoltVld"
  BMS_DSMR_FaultDspl/66(DSMR_BoardTempTmt) -> DSMR_BoardTempTmt/1  "DSMR_BoardTempTmt"
  BMS_DSMR_FaultDspl/67(DSMR_HvilMax) -> DSMR_HvilMax/1  "DSMR_HvilMax"
  BMS_DSMR_FaultDspl/68(DSMR_HvilMin) -> DSMR_HvilMin/1  "DSMR_HvilMin"
  BMS_DSMR_FaultDspl/69(DSMR_HvilSig) -> DSMR_HvilSig/1  "DSMR_HvilSig"
  BMS_DSMR_FaultDspl/70(DSMR_ChkSumMsg050Err) -> DSMR_ChkSumMsg050Err/1  "DSMR_ChkSumMsg050Err"
  BMS_DSMR_FaultDspl/71(DSMR_RcMsg050Mis) -> DSMR_RcMsg050Mis/1  "DSMR_RcMsg050Mis"
  BMS_DSMR_FaultDspl/72(DSMR_CrashHwNpl) -> DSMR_CrashHwNpl/1  "DSMR_CrashHwNpl"
  BMS_DSMR_FaultDspl/73(DSMR_IsoChkLv1) -> DSMR_IsoChkLv1/1  "DSMR_IsoChkLv1"
  BMS_DSMR_FaultDspl/74(DSMR_IsoChkLv2) -> DSMR_IsoChkLv2/1  "DSMR_IsoChkLv2"
  BMS_DSMR_FaultDspl/75(DSMR_InsResValdFault) -> DSMR_InsResValdFault/1  "DSMR_InsResValdFault"
  BMS_DSMR_FaultDspl/76(DSMR_Kl30OutRngErr) -> DSMR_Kl30OutRngErr/1  "DSMR_Kl30OutRngErr"
  BMS_DSMR_FaultDspl/77(DSMR_Kl30VoltLoErr) -> DSMR_Kl30VoltLoErr/1  "DSMR_Kl30VoltLoErr"
  BMS_DSMR_FaultDspl/78(DSMR_Kl30VoltHiErr) -> DSMR_Kl30VoltHiErr/1  "DSMR_Kl30VoltHiErr"
  BMS_DSMR_FaultDspl/79(DSMR_EepReadErr) -> DSMR_EepReadErr/1  "DSMR_EepReadErr"
  BMS_DSMR_FaultDspl/80(DSMR_BalStuckMax) -> DSMR_BalStuckMax/1  "DSMR_BalStuckMax"
  BMS_DSMR_FaultDspl/81(DSMR_BalStuckMin) -> DSMR_BalStuckMin/1  "DSMR_BalStuckMin"
  BMS_DSMR_FaultDspl/82(DSMR_CSCPwrSpyHiErr) -> DSMR_CSCPwrSpyHiErr/1  "DSMR_CSCPwrSpyHiErr"
  BMS_DSMR_FaultDspl/83(DSMR_CSCPwrSpyLoErr) -> DSMR_CSCPwrSpyLoErr/1  "DSMR_CSCPwrSpyLoErr"
  BMS_DSMR_FaultDspl/84(DSMR_CmcBordOTMax) -> DSMR_CmcBordOTMax/1  "DSMR_CmcBordOTMax"
  BMS_DSMR_FaultDspl/85(DSMR_BattTWarnMax) -> DSMR_BattTWarnMax/1  "DSMR_BattTWarnMax"
  BMS_DSMR_FaultDspl/86(DSMR_BattTWarnMin) -> DSMR_BattTWarnMin/1  "DSMR_BattTWarnMin"
  BMS_DSMR_FaultDspl/87(DSMR_BattTempVldMax) -> DSMR_BattTempVldMax/1  "DSMR_BattTempVldMax"
  BMS_DSMR_FaultDspl/88(DSMR_BattTHopMax) -> DSMR_BattTHopMax/1  "DSMR_BattTHopMax"
  BMS_DSMR_FaultDspl/89(DSMR_CellVoltRngHiErr) -> DSMR_CellVoltRngHiErr/1  "DSMR_CellVoltRngHiErr"
  BMS_DSMR_FaultDspl/90(DSMR_CellVoltRngLoErr) -> DSMR_CellVoltRngLoErr/1  "DSMR_CellVoltRngLoErr"
  BMS_DSMR_FaultDspl/91(DSMR_CellVoltWarnMax) -> DSMR_CellVoltWarnMax/1  "DSMR_CellVoltWarnMax"
  BMS_DSMR_FaultDspl/92(DSMR_CellVoltWarnMin) -> DSMR_CellVoltWarnMin/1  "DSMR_CellVoltWarnMin"
  BMS_DSMR_FaultDspl/93(DSMR_CellVoltVldMax) -> DSMR_CellVoltVldMax/1  "DSMR_CellVoltVldMax"
  BMS_DSMR_FaultDspl/94(DSMR_AChrgCurrMish) -> DSMR_AChrgCurrMish/1  "DSMR_AChrgCurrMish"
  BMS_DSMR_FaultDspl/95(DSMR_DChrgCurrMish) -> DSMR_DChrgCurrMish/1  "DSMR_DChrgCurrMish"
  BMS_DSMR_FaultDspl/96(DSMR_DChrgLowTempCurrMish) -> DSMR_DChrgLowTempCurrMish/1  "DSMR_DChrgLowTempCurrMish"
  BMS_DSMR_FaultDspl/97(DSMR_AChrgVoltMish) -> DSMR_AChrgVoltMish/1  "DSMR_AChrgVoltMish"
  BMS_DSMR_FaultDspl/98(DSMR_DChrgVoltMish) -> DSMR_DChrgVoltMish/1  "DSMR_DChrgVoltMish"
  BMS_DSMR_FaultDspl/99(DSMR_DChrgBattTMin) -> DSMR_DChrgBattTMin/1  "DSMR_DChrgBattTMin"
  BMS_DSMR_FaultDspl/100(DSMR_CC2Chk) -> DSMR_CC2Chk/1  "DSMR_CC2Chk"
  BMS_DSMR_FaultDspl/101(DSMR_APlusChk) -> DSMR_APlusChk/1  "DSMR_APlusChk"
  BMS_DSMR_FaultDspl/102(DSMR_DChrgMsgTmt) -> DSMR_DChrgMsgTmt/1  "DSMR_DChrgMsgTmt"
  BMS_DSMR_FaultDspl/103(DSMR_DChrgTNegElecMax) -> DSMR_DChrgTNegElecMax/1  "DSMR_DChrgTNegElecMax"
  BMS_DSMR_FaultDspl/104(DSMR_DChrgTNegElecMin) -> DSMR_DChrgTNegElecMin/1  "DSMR_DChrgTNegElecMin"
  BMS_DSMR_FaultDspl/105(DSMR_DChrgTNegElecSig) -> DSMR_DChrgTNegElecSig/1  "DSMR_DChrgTNegElecSig"
  BMS_DSMR_FaultDspl/106(DSMR_DChrgTPosElecMax) -> DSMR_DChrgTPosElecMax/1  "DSMR_DChrgTPosElecMax"
  BMS_DSMR_FaultDspl/107(DSMR_DChrgTPosElecMin) -> DSMR_DChrgTPosElecMin/1  "DSMR_DChrgTPosElecMin"
  BMS_DSMR_FaultDspl/108(DSMR_DChrgTPosElecSig) -> DSMR_DChrgTPosElecSig/1  "DSMR_DChrgTPosElecSig"
  BMS_DSMR_FaultDspl/109(DSMR_CcuSelfChkErr) -> DSMR_CcuSelfChkErr/1  "DSMR_CcuSelfChkErr"
  BMS_DSMR_FaultDspl/110(DSMR_ChrgOCMin) -> DSMR_ChrgOCMin/1  "DSMR_ChrgOCMin"
  BMS_DSMR_FaultDspl/111(DSMR_ChrgOCMax) -> DSMR_ChrgOCMax/1  "DSMR_ChrgOCMax"
  BMS_DSMR_FaultDspl/112(DSMR_DisChOCMin) -> DSMR_DisChOCMin/1  "DSMR_DisChOCMin"
  BMS_DSMR_FaultDspl/113(DSMR_DisChOCMax) -> DSMR_DisChOCMax/1  "DSMR_DisChOCMax"
  BMS_DSMR_FaultDspl/114(DSMR_SocRngLoMax) -> DSMR_SocRngLoMax/1  "DSMR_SocRngLoMax"
  BMS_DSMR_FaultDspl/115(DSMR_SocRngLoMin) -> DSMR_SocRngLoMin/1  "DSMR_SocRngLoMin"
  BMS_DSMR_FaultDspl/116(DSMR_SocRngHiMax) -> DSMR_SocRngHiMax/1  "DSMR_SocRngHiMax"
  BMS_DSMR_FaultDspl/117(DSMR_SocRngHiMin) -> DSMR_SocRngHiMin/1  "DSMR_SocRngHiMin"
  BMS_DSMR_FaultDspl/118(DSMR_InClntOverTmp) -> DSMR_InClntOverTmp/1  "DSMR_InClntOverTmp"
  BMS_DSMR_FaultDspl/119(DSMR_OutClntOverTmp) -> DSMR_OutClntOverTmp/1  "DSMR_OutClntOverTmp"
  BMS_DSMR_FaultDspl/120(DSMR_ClntDsTElecMax) -> DSMR_ClntDsTElecMax/1  "DSMR_ClntDsTElecMax"
  BMS_DSMR_FaultDspl/121(DSMR_ClntDsTElecMin) -> DSMR_ClntDsTElecMin/1  "DSMR_ClntDsTElecMin"
  BMS_DSMR_FaultDspl/122(DSMR_ClntDsTElecSig) -> DSMR_ClntDsTElecSig/1  "DSMR_ClntDsTElecSig"
  BMS_DSMR_FaultDspl/123(DSMR_ClntUsTElecMax) -> DSMR_ClntUsTElecMax/1  "DSMR_ClntUsTElecMax"
  BMS_DSMR_FaultDspl/124(DSMR_ClntUsTElecMin) -> DSMR_ClntUsTElecMin/1  "DSMR_ClntUsTElecMin"
  BMS_DSMR_FaultDspl/125(DSMR_ClntUsTElecSig) -> DSMR_ClntUsTElecSig/1  "DSMR_ClntUsTElecSig"
  BMS_DSMR_FaultDspl/126(DSMR_CoolPerfPlaus) -> DSMR_CoolPerfPlaus/1  "DSMR_CoolPerfPlaus"
  BMS_DSMR_FaultDspl/127(DSMR_HtgPerfPlaus) -> DSMR_HtgPerfPlaus/1  "DSMR_HtgPerfPlaus"
  BMS_DSMR_FaultDspl/128(DSMR_DChrgFobd) -> DSMR_DChrgFobd/1  "DSMR_DChrgFobd"
  BMS_DSMR_FaultDspl/129(DSMR_DChrgHvOnFail) -> DSMR_DChrgHvOnFail/1  "DSMR_DChrgHvOnFail"
  BMS_DSMR_FaultDspl/130(DSMR_AChgHVOnTmt) -> DSMR_AChgHVOnTmt/1  "DSMR_AChgHVOnTmt"
  BMS_DSMR_FaultDspl/131(DSMR_AChgHVOffTmt) -> DSMR_AChgHVOffTmt/1  "DSMR_AChgHVOffTmt"
  BMS_DSMR_FaultDspl/132(DSMR_AChgS2ClsdTmt) -> DSMR_AChgS2ClsdTmt/1  "DSMR_AChgS2ClsdTmt"
  BMS_DSMR_FaultDspl/133(DSMR_DChrgStakeErr) -> DSMR_DChrgStakeErr/1  "DSMR_DChrgStakeErr"
  BMS_DSMR_FaultDspl/134(DSMR_DChrgStkVoltErr) -> DSMR_DChrgStkVoltErr/1  "DSMR_DChrgStkVoltErr"
  BMS_DSMR_FaultDspl/135(DSMR_DChrgStkCurrErr) -> DSMR_DChrgStkCurrErr/1  "DSMR_DChrgStkCurrErr"
  BMS_DSMR_FaultDspl/136(DSMR_AChgPileRdyTmt) -> DSMR_AChgPileRdyTmt/1  "DSMR_AChgPileRdyTmt"
  BMS_DSMR_FaultDspl/137(DSMR_DChrgCHMTmt) -> DSMR_DChrgCHMTmt/1  "DSMR_DChrgCHMTmt"
  BMS_DSMR_FaultDspl/138(DSMR_DChrgCRMTmt) -> DSMR_DChrgCRMTmt/1  "DSMR_DChrgCRMTmt"
  BMS_DSMR_FaultDspl/139(DSMR_DChrgCMLTmt) -> DSMR_DChrgCMLTmt/1  "DSMR_DChrgCMLTmt"
  BMS_DSMR_FaultDspl/140(DSMR_DChrgCROTmt) -> DSMR_DChrgCROTmt/1  "DSMR_DChrgCROTmt"
  BMS_DSMR_FaultDspl/141(DSMR_DChrgCCSTmt) -> DSMR_DChrgCCSTmt/1  "DSMR_DChrgCCSTmt"
  BMS_DSMR_FaultDspl/142(DSMR_DChrgCSTTmt) -> DSMR_DChrgCSTTmt/1  "DSMR_DChrgCSTTmt"
  BMS_DSMR_FaultDspl/143(DSMR_DChrgCSDTmt) -> DSMR_DChrgCSDTmt/1  "DSMR_DChrgCSDTmt"
  BMS_DSMR_FaultDspl/144(DSMR_DChrgParaChk) -> DSMR_DChrgParaChk/1  "DSMR_DChrgParaChk"
  BMS_DSMR_FaultDspl/145(DSMR_DChrgCableChk) -> DSMR_DChrgCableChk/1  "DSMR_DChrgCableChk"
  BMS_DSMR_FaultDspl/146(DSMR_DChrgSLACTOut) -> DSMR_DChrgSLACTOut/1  "DSMR_DChrgSLACTOut"
  BMS_DSMR_FaultDspl/147(DSMR_DChrgCnntErr) -> DSMR_DChrgCnntErr/1  "DSMR_DChrgCnntErr"
  BMS_DSMR_FaultDspl/148(DSMR_DChrgLckErr) -> DSMR_DChrgLckErr/1  "DSMR_DChrgLckErr"
  BMS_DSMR_FaultDspl/149(DSMR_AChrgCnntErr) -> DSMR_AChrgCnntErr/1  "DSMR_AChrgCnntErr"
  BMS_DSMR_FaultDspl/150(DSMR_AChgLckTmt) -> DSMR_AChgLckTmt/1  "DSMR_AChgLckTmt"
  BMS_DSMR_FaultDspl/151(DSMR_AChgRdyPndiTmt) -> DSMR_AChgRdyPndiTmt/1  "DSMR_AChgRdyPndiTmt"
  BMS_DSMR_FaultDspl/152(DSMR_AChgRdyTmt) -> DSMR_AChgRdyTmt/1  "DSMR_AChgRdyTmt"
  BMS_DSMR_FaultDspl/153(DSMR_AChgingErr) -> DSMR_AChgingErr/1  "DSMR_AChgingErr"
  BMS_DSMR_FaultDspl/154(DSMR_AChgUnlckTmt) -> DSMR_AChgUnlckTmt/1  "DSMR_AChgUnlckTmt"
  BMS_DSMR_FaultDspl/155(DSMR_AChgFobd) -> DSMR_AChgFobd/1  "DSMR_AChgFobd"
  BMS_DSMR_FaultDspl/156(DSMR_SocValJmp) -> DSMR_SocValJmp/1  "DSMR_SocValJmp"
